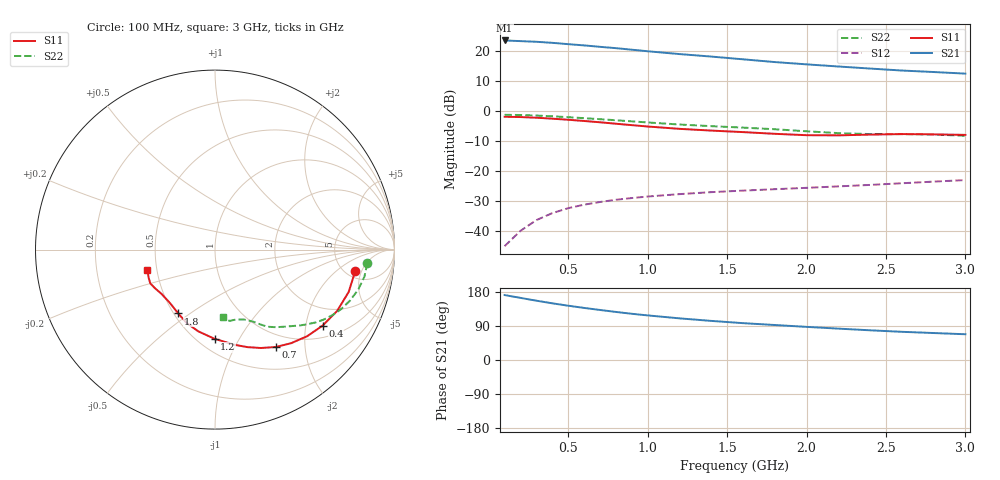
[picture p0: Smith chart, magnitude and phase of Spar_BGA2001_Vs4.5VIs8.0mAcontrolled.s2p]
! Filename: 4_58G1.001
! Title: BGA2001 X0297-20 HFE=80
! Bias: Vce=4.5V; Ic=8.0mA controlled / noise data included
! Company: NXP Semiconductors NL
! User: Quality&Reliability T&D
! Measure time: 23 Oct 1998 / 08:34:37
#  MHz  S  MA  R 50
! Freq  S11  S21  S12  S22  :
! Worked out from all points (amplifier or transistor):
!   20 points, 100 MHz to 3 GHz, reference 50 ohm
!   highest |S21| = 23.4 dB at 100 MHz (marker M1)
!   |S21| within 3 dB of that: start of sweep to 883.8 MHz
!   unconditionally stable (mu >= 1): 1.819 GHz to end of sweep
!   at 400 MHz: K = 0.40, MSG = 28.4 dB, |S12| = -34.2 dB
!   at 1.2 GHz: K = 0.72, MSG = 23.4 dB, |S12| = -27.9 dB
!   at 3 GHz: K = 1.26, MAG = 14.7 dB, |S12| = -23.2 dB
!   lowest NFmin = 1.57 dB at 1.8 GHz
!   S11 on the Smith chart (normalised r, x): 100 MHz: 6.01, -3.86; 400 MHz: 1.36, -2.50; 700 MHz: 0.81, -1.48; 1.2 GHz: 0.60, -0.79; 1.8 GHz: 0.53, -0.45; 3 GHz: 0.44, -0.12
100  0.7903 -8.8  14.81 171.4  0.005485 59.5  0.8519 -5.1
200  0.7814 -17.5  14.44 163.9  0.009902 70.2  0.846 -10.3
300  0.7616 -26.6  14.07 156.5  0.01491 71.0  0.8283 -15.7
400  0.7342 -35.2  13.52 149.6  0.01951 68.7  0.8043 -20.6
500  0.7046 -43.2  12.85 143.3  0.02359 66.3  0.7777 -25.2
600  0.672 -50.9  12.25 137.4  0.02698 63.7  0.749 -29.2
700  0.6396 -58.0  11.6 132.1  0.02993 61.5  0.7206 -32.8
800  0.6048 -65.0  11.03 126.8  0.03259 59.6  0.6915 -35.9
900  0.5731 -71.5  10.38 122.0  0.0348 58.1  0.6627 -38.8
1000  0.5435 -77.9  9.785 117.7  0.0369 57.1  0.6353 -41.7
1200  0.497 -90.3  8.78 109.9  0.04048 55.5  0.5867 -46.9
1400  0.4647 -101.6  7.98 103.2  0.04369 54.8  0.5511 -51.7
1600  0.4386 -111.0  7.18 97.2  0.04633 55.1  0.5212 -55.6
1800  0.4107 -119.9  6.46 92.3  0.04892 56.3  0.4893 -58.6
2000  0.3894 -130.0  5.914 87.4  0.05155 56.9  0.4527 -62.2
2200  0.3868 -140.2  5.449 82.8  0.05449 57.2  0.4217 -67.5
2400  0.3983 -147.6  5.035 78.4  0.05767 58.2  0.4065 -73.5
2600  0.4067 -152.4  4.666 74.4  0.06147 59.8  0.4054 -78.2
2800  0.4017 -156.9  4.406 71.2  0.06549 60.4  0.3998 -80.8
3000  0.3941 -162.9  4.143 68.0  0.06943 61.1  0.3799 -83.4
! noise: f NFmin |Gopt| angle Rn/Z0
900  1.61  0.23  21.6  0.31
1000  1.67  0.2  19.6  0.28
1800  1.575  0.204  73.63  0.262
2000  1.625  0.169  75.08  0.221
2200  1.728  0.141  83.15  0.222
2400  1.775  0.156  107.3  0.223
